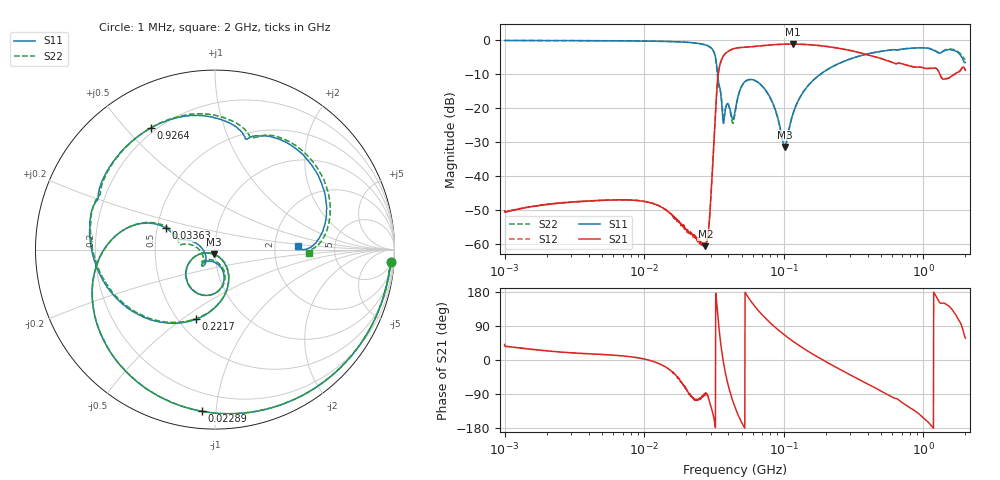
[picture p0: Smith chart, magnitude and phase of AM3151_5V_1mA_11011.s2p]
! Date/Time: Fri Jun 26 11:08:01 2020
! Network Analyzer:  Rev:
! Sweep from 1000000.0 to 2000000000.0, 1601 Points ! Power Supply: 0 V, 0 A
# HZ S DB R 50
!freq MagS11 AngS11 MagS21 AngS21 MagS12 AngS12 MagS22 AngS22
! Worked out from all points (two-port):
!   1601 points, 1 MHz to 2 GHz, reference 50 ohm
!   highest |S21| = -1.22 dB at 115.6 MHz (marker M1); lowest = -60.5 dB at 27.42 MHz (marker M2)
!   |S21| within 3 dB of the highest: 37.71 MHz to 386.3 MHz (348.5 MHz wide, 164 % of centre)
!   lowest |S11| = -31.4 dB at 101.7 MHz (marker M3), VSWR 1.06, Z = 49.1 - j2.51 ohm
!   |S11| at or under -10 dB: 33.53 MHz to 183.7 MHz (150.1 MHz wide, 138 % of centre)
!   |S22| runs from -32.0 to -0.2 dB; largest |S21 - S12| = 0.0084
!   S11 on the Smith chart (normalised r, x): 1 MHz: 7, -27; 22.89 MHz: 0.09, -0.92; 33.63 MHz: 0.56, +0.15; 221.7 MHz: 0.61, -0.57; 926.4 MHz: 0.18, +0.59; 2 GHz: 2.73, +0.15
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1000000  -0.16 -4.0  -50.14 41.0  -50.53 36.8  -0.16 -4.0
3555161  -0.22 -13.5  -47.36 17.6  -47.41 17.4  -0.21 -13.4
1.263916e7  -0.38 -48.1  -48.62 -8.7  -48.62 -9.1  -0.40 -48.1
2.288819e7  -0.88 -94.8  -57.59 -103.7  -57.53 -102.9  -0.89 -94.9
2.741642e7  -1.45 -124.1  -60.50 -88.0  -60.08 -89.0  -1.47 -124.5
2.944137e7  -2.00 -142.6  -52.08 -110.9  -51.92 -111.9  -2.03 -143.4
3.362991e7  -10.51 156.3  -11.50 121.4  -11.49 121.3  -11.64 156.5
3.526606e7  -15.38 161.4  -6.57 45.8  -6.57 45.7  -15.28 169.6
3.751269e7  -22.88 -133.8  -4.32 -19.8  -4.32 -19.8  -21.84 -141.7
4.086156e7  -19.74 -132.2  -3.11 -79.7  -3.11 -79.8  -20.14 -137.1
4.493426e7  -20.54 -74.6  -2.45 -126.5  -2.45 -126.6  -21.04 -71.2
5.206369e7  -12.45 -88.1  -2.14 -177.3  -2.15 -177.3  -12.52 -87.1
6.477976e7  -12.31 -128.7  -1.83 133.1  -1.82 133.1  -12.38 -128.4
8.293223e7  -18.26 -160.5  -1.42 92.6  -1.43 92.5  -18.42 -160.7
1.017274e8  -31.44 -107.8  -1.25 65.3  -1.24 65.2  -31.93 -105.2
1.156494e8  -22.02 -55.3  -1.22 50.1  -1.23 50.1  -22.02 -53.8
1.589914e8  -12.20 -75.7  -1.46 16.9  -1.45 16.8  -12.23 -75.7
2.217143e8  -7.89 -105.3  -2.12 -13.4  -2.13 -13.6  -7.93 -105.9
5.652395e8  -3.00 170.3  -6.24 -93.3  -6.20 -93.4  -3.01 168.3
9.264031e8  -2.31 117.7  -7.97 -141.7  -7.99 -141.7  -2.29 115.4
1.461712e9  -2.95 59.8  -11.39 146.6  -11.28 146.5  -2.78 58.0
2e9  -6.64 2.7  -8.87 57.6  -9.02 57.2  -5.66 -1.9
